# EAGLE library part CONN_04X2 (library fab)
Multi connection point. Often used as Generic Header-pin footprint for 0.1 inch spaced/style header connections On any of the 0.1 inch spaced packages, you can populate with these: Break Away Headers - Straight (PRT-00116) Break Away Male Headers - Right Angle (PRT-00553) Female Headers (PRT-00115) Break Away Headers - Machine Pin (PRT-00117) Break Away Female Headers - Swiss Machine Pin (PRT-00743)
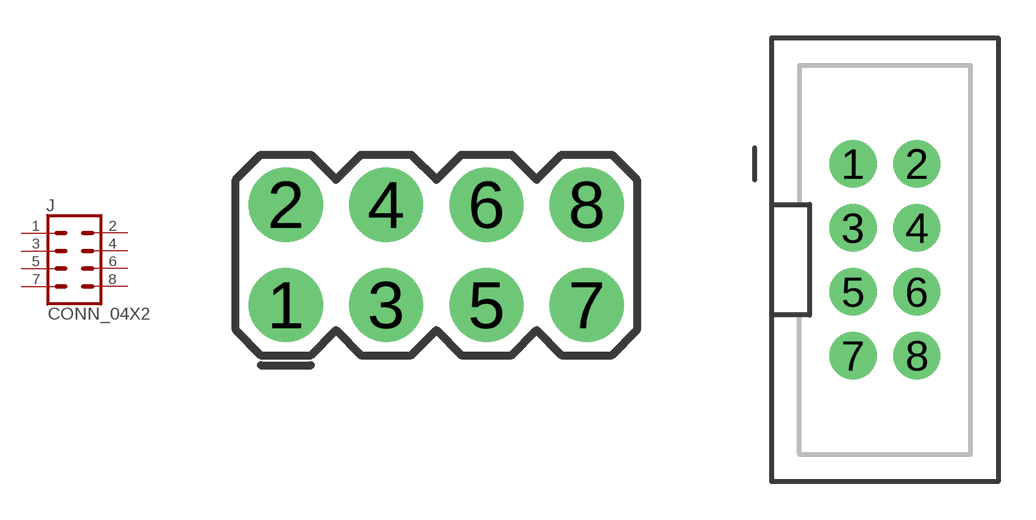
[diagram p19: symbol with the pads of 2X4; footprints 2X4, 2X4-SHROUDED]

Designator prefix J

## CONN_04X2  [2X4]
1  1  pas
2  2  pas
3  3  pas
4  4  pas
5  5  pas
6  6  pas
7  7  pas
8  8  pas

## CONN_04X2SHROUDED  [2X4-SHROUDED]
Pads as for 2X4

## CONN_04X2SHROUDED-SQUISH  [2X4-SHROUDED-SQUISH]
Pads as for 2X4

## Footprint 2X4 (pad centres in mm)
Plated Through Hole - 2x4 Specifications: Pin count:8 Pin pitch:0.1" Example device(s): CONN_04x2
drill 1.016 pad 1.88: 1 -3.81,-1.27; 2 -3.81,1.27; 3 -1.27,-1.27; 4 -1.27,1.27; 5 1.27,-1.27; 6 1.27,1.27; 7 3.81,-1.27; 8 3.81,1.27

## Footprint 2X4-SHROUDED (pad centres in mm)
Plated Through Hole - 2x3 Shrouded Header Specifications: Pin count:6 Pin pitch:0.1" Datasheet referenced for footprint Example device(s): CONN_03x2
drill 1.016 pad 1.88: 1 -1.27,2.54; 2 1.27,2.54; 3 -1.27,0; 4 1.27,0; 5 -1.27,-2.54; 6 1.27,-2.54; 7 -1.27,-5.08; 8 1.27,-5.08

## Footprint 2X4-SHROUDED-SQUISH (pad centres in mm)
Plated Through Hole - 2x3 Shrouded Header Specifications: Pin count:6 Pin pitch:0.1" Datasheet referenced for footprint Example device(s): CONN_03x2
drill 1.016 pad 1.676: 1 -1.27,2.54; 2 1.27,2.54; 3 -1.27,0; 4 1.27,0; 5 -1.27,-2.54; 6 1.27,-2.54; 7 -1.27,-5.08; 8 1.27,-5.08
